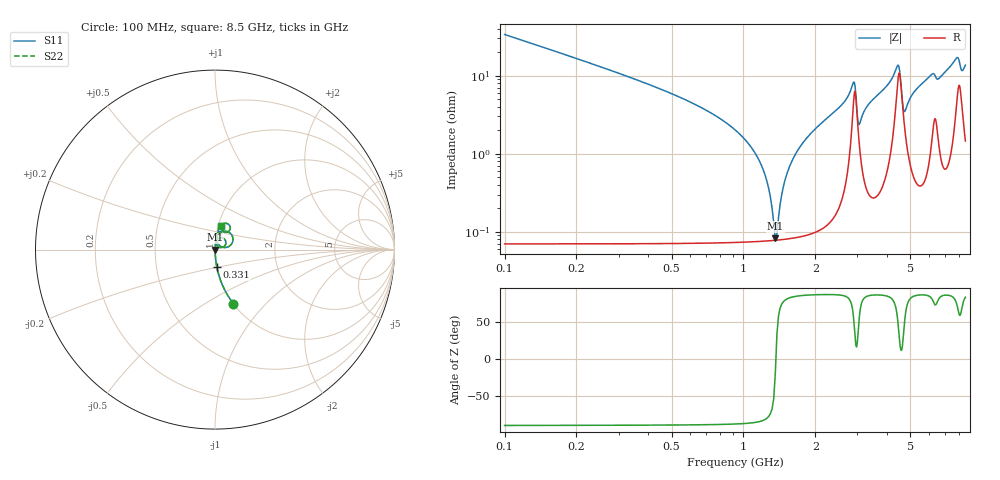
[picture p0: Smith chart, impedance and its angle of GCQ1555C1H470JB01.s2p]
!Murata Part Number: GCQ1555C1H470JB01
!These Parameters are Measured in Series Mode Connection
!Data Generated on Jan 08, 2026
!  o--ll--o
!Port1  Port2
!  o------o
!Operation Temp=25[degC], DC Bias Voltage=0[V]
!Freq. Start=100[MHz] Stop=9[GHz] 401[Steps]
# Hz S RI R 50
!Freq.(Hz) S11(Real) S11(Imag) S21(Real) S21(Imag) S12(Real) S12(Imag) S22(Real) S22(Imag)
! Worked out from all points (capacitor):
!   401 points, 100 MHz to 8.5 GHz, reference 50 ohm
!   read as one part in series: C = 47 pF near 142 MHz
!   lowest |Z| = 82.5 mohm at 1.36 GHz (marker M1)
!   series resonance near 1.367 GHz, so ESL is about 290 pH
!   S11 on the Smith chart (normalised r, x): 100 MHz: 1.00, -0.67; 331 MHz: 1.00, -0.19; 8.5 GHz: 1.03, +0.27
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1e8  0.1024 -0.3021  0.8976 0.3021  0.8976 0.3021  0.1024 -0.3021
3.31e8  0.0099 -0.0954  0.9901 0.0954  0.9901 0.0954  0.0099 -0.0954
1.108e9  0.00086 -0.0107  0.9991 0.0107  0.9991 0.0107  0.00086 -0.0107
1.234e9  0.000788 -0.00519  0.9992 0.00519  0.9992 0.00519  0.000788 -0.00519
1.36e9  0.000779 -0.000269  0.9992 0.000269  0.9992 0.000269  0.000779 -0.000269
1.402e9  0.000787 0.00128  0.9992 -0.00128  0.9992 -0.00128  0.000787 0.00128
1.507e9  0.00083 0.00499  0.9992 -0.00499  0.9992 -0.00499  0.00083 0.00499
1.654e9  0.000938 0.0099  0.9991 -0.0099  0.9991 -0.0099  0.000938 0.0099
1.864e9  0.00119 0.0166  0.9988 -0.0166  0.9988 -0.0166  0.00119 0.0166
2.914e9  0.0592 0.0496  0.9408 -0.0496  0.9408 -0.0496  0.0592 0.0496
3.019e9  0.0208 0.0137  0.9792 -0.0137  0.9792 -0.0137  0.0208 0.0137
3.061e9  0.0127 0.02  0.9873 -0.02  0.9873 -0.02  0.0127 0.02
3.334e9  0.00486 0.0421  0.9951 -0.0421  0.9951 -0.0421  0.00486 0.0421
4.3e9  0.0377 0.0991  0.9623 -0.0991  0.9623 -0.0991  0.0377 0.0991
4.468e9  0.0992 0.0684  0.9008 -0.0684  0.9008 -0.0684  0.0992 0.0684
4.72e9  0.0233 0.0246  0.9767 -0.0246  0.9767 -0.0246  0.0233 0.0246
5.119e9  0.0087 0.0576  0.9913 -0.0576  0.9913 -0.0576  0.0087 0.0576
5.707e9  0.0111 0.0822  0.9889 -0.0822  0.9889 -0.0822  0.0111 0.0822
7.114e9  0.02 0.1146  0.98 -0.1146  0.98 -0.1146  0.02 0.1146
7.828e9  0.0672 0.1453  0.9328 -0.1453  0.9328 -0.1453  0.0672 0.1453
8.206e9  0.0516 0.0983  0.9484 -0.0983  0.9484 -0.0983  0.0516 0.0983
8.5e9  0.0316 0.1294  0.9684 -0.1294  0.9684 -0.1294  0.0316 0.1294
